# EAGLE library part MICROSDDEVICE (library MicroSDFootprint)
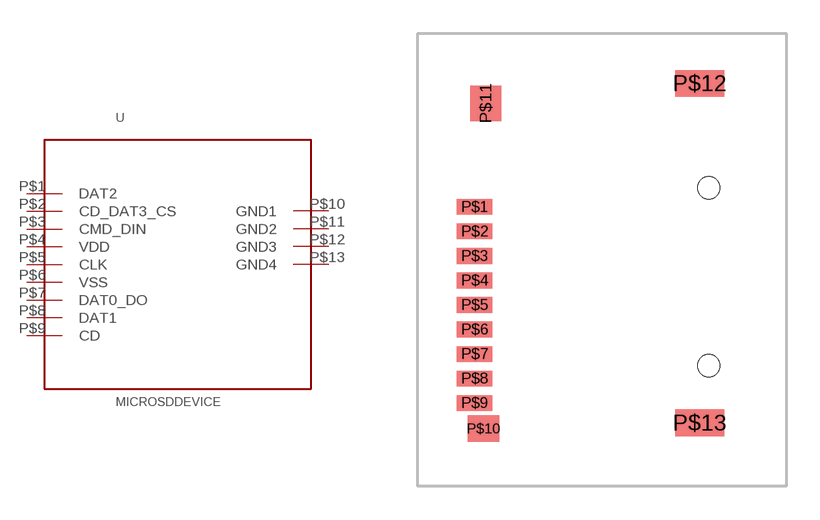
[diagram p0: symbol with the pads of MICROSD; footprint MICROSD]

Designator prefix -

## MICROSDDEVICE  [MICROSD]
P$1  DAT2
P$2  CD_DAT3_CS
P$3  CMD_DIN
P$4  VDD
P$5  CLK
P$6  VSS
P$7  DAT0_DO
P$8  DAT1
P$9  CD
P$10  GND1
P$11  GND2
P$12  GND3
P$13  GND4

## Footprint MICROSD (pad centres in mm)
smd 1.6 x 0.7: P$1 -3.81,1.1; P$2 -3.81,0; P$3 -3.81,-1.1; P$4 -3.81,-2.2; P$5 -3.81,-3.3; P$6 -3.81,-4.4; P$7 -3.81,-5.5; P$8 -3.81,-6.6; P$9 -3.81,-7.7
smd 1.4 x 1.2: P$10 -3.41,-8.85
smd 1.4 x 1.6: P$11 -3.31,5.75
smd 2.2 x 1.2: P$12 6.29,6.65; P$13 6.29,-8.59
hole 1 at 6.69,1.95
hole 1 at 6.69,-6.03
